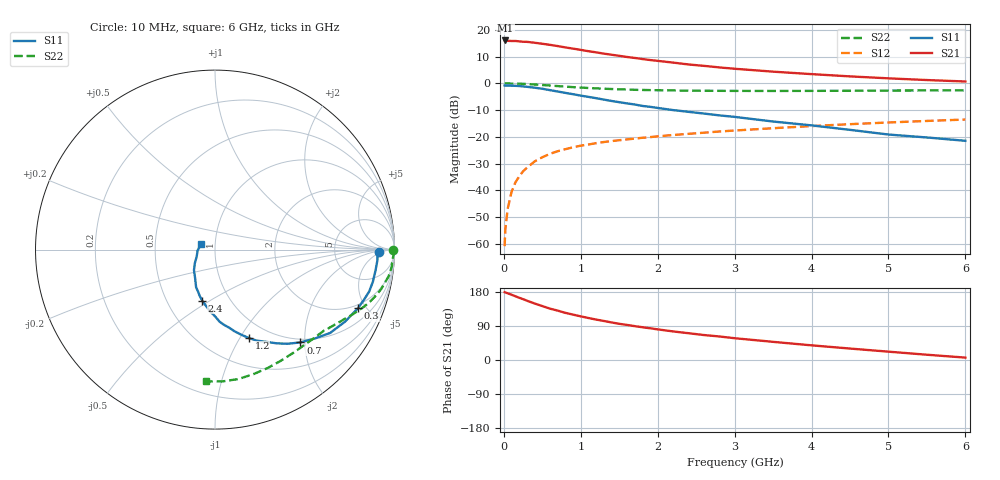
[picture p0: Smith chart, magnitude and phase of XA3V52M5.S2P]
! SIEMENS Discrete & RF Semiconductors
! BFY180
! Si NPN RF Bipolar Junction Transistor in MICRO-X
! VCE = 3.5 V  IC = 2.5 mA
! Common Emitter S-Parameters:  May  1997
# GHz  S  MA  R  50
!  f  S11  S21  S12  S22
! GHz  MAG  ANG  MAG  ANG  MAG  ANG  MAG  ANG
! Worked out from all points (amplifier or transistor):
!   36 points, 10 MHz to 6 GHz, reference 50 ohm
!   highest |S21| = 16.0 dB at 20 MHz (marker M1)
!   |S21| within 3 dB of that: start of sweep to 888 MHz
!   unconditionally stable (mu >= 1): 2.5 GHz to end of sweep
!   at 250 MHz: K = 0.15, MSG = 24.2 dB, |S12| = -32.9 dB
!   at 1.4 GHz: K = 0.74, MSG = 16.2 dB, |S12| = -21.6 dB
!   at 6 GHz: K = 1.07, MAG = 5.6 dB, |S12| = -13.5 dB
!   S11 on the Smith chart (normalised r, x): 10 MHz: 21, -3; 300 MHz: 1.75, -4.41; 700 MHz: 0.93, -1.91; 1.2 GHz: 0.80, -1.09; 2.4 GHz: 0.74, -0.46; 6 GHz: 0.85, +0.05
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0.01  0.9126 -0.8  6.225 178.9  0.0009 75.4  0.9945 -0.2
0.02  0.9052 -1.6  6.334 178.1  0.0019 96.7  0.9977 -0.7
0.05  0.907 -3.6  6.224 176.1  0.0045 86.4  0.9954 -1.8
0.1  0.9019 -7.4  6.195 172.2  0.0093 84.7  0.9894 -3.7
0.15  0.8977 -11.5  6.191 168.2  0.014 82.2  0.9896 -5.4
0.3  0.8609 -22.3  5.967 156.5  0.0264 76.8  0.9681 -10.4
0.4  0.8282 -29.0  5.739 149.1  0.0346 72.3  0.9509 -13.5
0.5  0.792 -35.9  5.497 142.3  0.0414 68.5  0.9293 -16.3
0.6  0.7455 -41.6  5.241 135.5  0.048 65.6  0.9089 -18.8
0.7  0.7025 -47.4  4.973 130.3  0.0537 62.8  0.8878 -21.1
0.8  0.6622 -52.4  4.688 124.4  0.0587 60.4  0.8669 -23.1
1.1  0.5577 -65.4  3.986 110.8  0.0717 54.5  0.8175 -28.3
1.2  0.5272 -69.1  3.795 106.7  0.076 53.0  0.805 -29.9
1.5  0.4437 -79.5  3.269 95.5  0.0863 49.6  0.7727 -34.2
1.7  0.4022 -86.4  2.988 89.4  0.0924 48.1  0.7562 -36.7
2.2  0.316 -99.4  2.442 75.4  0.108 44.3  0.7358 -43.3
2.4  0.2928 -104.1  2.253 70.7  0.1135 42.9  0.7297 -45.9
3  0.2356 -116.5  1.873 57.5  0.1309 39.2  0.7215 -53.3
3.5  0.193 -125.1  1.652 47.9  0.1447 36.1  0.7198 -59.7
4.5  0.1348 -146.3  1.348 30.2  0.1722 28.9  0.7261 -72.8
5.5  0.0971 -176.7  1.151 13.9  0.1979 21.3  0.7356 -86.8
6  0.0841 158.4  1.082 6.3  0.2102 17.0  0.7366 -94.0
